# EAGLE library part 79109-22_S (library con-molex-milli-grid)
RECEPTACAL
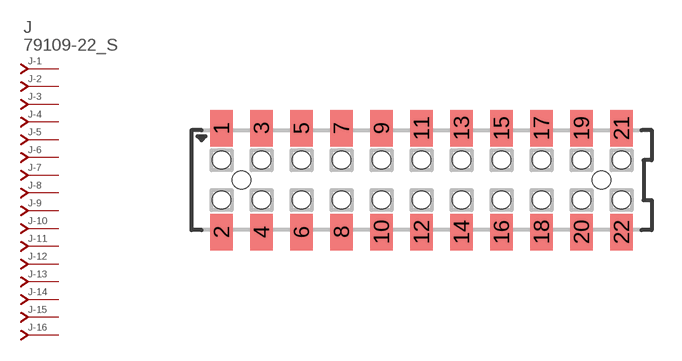
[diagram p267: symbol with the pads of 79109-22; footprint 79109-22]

Designator prefix J; gates -1=J-NV -2=J-N -3=J-N -4=J-N -5=J-N -6=J-N -7=J-N -8=J-N -9=J-N -10=J-N -11=J-N -12=J-N -13=J-N -14=J-N -15=J-N -16=J-N -17=J-N -18=J-N -19=J-N -20=J-N -21=J-N -22=J-N

## 79109-22_S  [79109-22]
1  -1:J  pas
2  -2:J  pas
3  -3:J  pas
4  -4:J  pas
5  -5:J  pas
6  -6:J  pas
7  -7:J  pas
8  -8:J  pas
9  -9:J  pas
10  -10:J  pas
11  -11:J  pas
12  -12:J  pas
13  -13:J  pas
14  -14:J  pas
15  -15:J  pas
16  -16:J  pas
17  -17:J  pas
18  -18:J  pas
19  -19:J  pas
20  -20:J  pas
21  -21:J  pas
22  -22:J  pas

## Footprint 79109-22 (pad centres in mm)
RECEPTACAL SMD Dual Row, Vertical, Pass-Thru
smd 1.12 x 1.83: 1 -10,2.6; 2 -10,-2.6; 3 -8,2.6; 4 -8,-2.6; 5 -6,2.6; 6 -6,-2.6; 7 -4,2.6; 8 -4,-2.6; 9 -2,2.6; 10 -2,-2.6; 11 0,2.6; 12 0,-2.6; 13 2,2.6; 14 2,-2.6; 15 4,2.6; 16 4,-2.6; 17 6,2.6; 18 6,-2.6; 19 8,2.6; 20 8,-2.6; 21 10,2.6; 22 10,-2.6
hole 0.914 at -9,0
hole 0.914 at -10,1
hole 0.914 at -10,-1
hole 0.914 at -8,-1
hole 0.914 at -8,1
hole 0.914 at -6,-1
hole 0.914 at -6,1
hole 0.914 at 9,0
hole 0.914 at -4,1
hole 0.914 at -4,-1
hole 0.914 at -2,1
hole 0.914 at -2,-1
hole 0.914 at 0,1
hole 0.914 at 0,-1
hole 0.914 at 2,1
hole 0.914 at 2,-1
hole 0.914 at 4,-1
hole 0.914 at 4,1
hole 0.914 at 6,1
hole 0.914 at 6,-1
hole 0.914 at 8,1
hole 0.914 at 8,-1
hole 0.914 at 10,1
hole 0.914 at 10,-1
